| TEXAS INSTRUMENTS INCORPORATED
| Standard Linear and Logic Group
| IBIS Model of SN74ACT244
| OCTAL BUFFERS/DRIVERS WITH 3-STATE OUTPUTS
| This file contains package information for the following:
|  SSOP 20-pin (DB) package as [Component] ACT244A_DB
|  SOIC 20-pin (DW) package as [Component] ACT244A_DW
|  PDIP 20-pin (N) package as [Component] ACT244A_N
|  SOP 20-pin (NS) package as [Component] ACT244A_NS
|  TSSOP 20-pin (PW) package as [Component] ACT244A_PW
| This device can be powered at the following Vccs:
|  5 volt Vcc
| This file provides unique models under the [Model Selector] for each Vcc.
| For operation at a specific Vcc, select the appropriate model after each
| [Model Selector] keyword.
[IBIS Ver]   3.2
[Comment char]  |_char
[File Name]   sn74act244.ibs
[File Rev]   1.2 | a_die
[Date]   September 02, 2003
[Source]   Data created from TI-SPICE simulations at TI-SLL.
[Notes]   The following is an IBIS list for the ACT244A.
   Please contact sllibis@ti.com with questions and
   comments concerning SLL IBIS models.
   This IBIS model is created from a BA (back annotated netlist)
[Disclaimer] Property of Texas Instruments Incorporated.  Unauthorized
   reproduction and/or distribution is strictly prohibited.
   This product is protected under copyright law.
   Created  2003, (C) Copyright  2003, Texas Instruments
   Incorporated, All Rights Reserved
   UNLESS THERE IS A SIGNED, WRITTEN AGREEMENT TO THE
   CONTRARY, TEXAS INSTRUMENTS (TI) IS PROVIDING THE IBIS
   MODELS  AND WITHOUT ANY WARRANTY, EXPRESSED OR
   IMPLIED.  TI assumes no liability for:
   1) the accuracy of the IBIS models provided to your
   company;
   2) the proper functioning of these IBIS Models in your
   design or for any resulting applications; or
   3) infringement of patents, copyrights or intellectual
   property rights resulting from your use of these IBIS
   models.
   TI provides IBIS Models as a service to our customers.
   You and your company shall not distribute, sell or give
   these models to anyone else without prior written
   permission from TI.
   TI reserves the right to make changes to our products or
   to discontinue any semiconductor product or service
   without notice, and advises our customers to obtain the
   latest version of relevant information to verify, before
   placing orders, that the information being relied on is
   current.
   Please be aware that your receipt and use of the IBIS
   information provided shall serve as acceptance of these
   terms and conditions.  If you do not accept these terms,
   you should return or destroy the IBIS models and any
   other accompanying information immediately.
| Component ACT244A_DB 20-pin SSOP
[Component]   ACT244A_DB
[Manufacturer]   Texas Instruments, Inc.
[Package]
|   typ   min   max
R_pkg   4.000e-02   3.500e-02   5.100e-02
L_pkg   3.495e-09   3.035e-09   4.314e-09
C_pkg   4.200e-13   3.460e-13   5.020e-13
[Pin]   signal_name   model_name   R_pin   L_pin   C_pin
1   1NOE   ACT244_NOE   4.900e-02   4.310e-09   5.020e-13
2   1A1   ACT244_IN   4.800e-02   3.903e-09   4.870e-13
3   2Y4   ACT244_OUT   3.500e-02   3.189e-09   3.960e-13
4   1A2   ACT244_IN   3.500e-02   3.036e-09   3.470e-13
5   2Y3   ACT244_OUT   3.500e-02   3.035e-09   3.670e-13
6   1A3   ACT244_IN   3.500e-02   3.035e-09   3.670e-13
7   2Y2   ACT244_OUT   3.500e-02   3.036e-09   3.470e-13
8   1A4   ACT244_IN   3.500e-02   3.189e-09   3.970e-13
9   2Y1   ACT244_OUT   4.700e-02   3.899e-09   4.880e-13
10   GND   GND   5.100e-02   4.314e-09   5.000e-13
11   2A1   ACT244_IN   5.100e-02   4.314e-09   5.000e-13
12   1Y4   ACT244_OUT   4.700e-02   3.899e-09   4.880e-13
13   2A2   ACT244_IN   3.500e-02   3.189e-09   3.970e-13
14   1Y3   ACT244_OUT   3.500e-02   3.036e-09   3.460e-13
15   2A3   ACT244_IN   3.500e-02   3.035e-09   3.670e-13
16   1Y2   ACT244_OUT   3.500e-02   3.035e-09   3.670e-13
17   2A4   ACT244_IN   3.500e-02   3.036e-09   3.460e-13
18   1Y1   ACT244_OUT   3.500e-02   3.189e-09   3.970e-13
19   2NOE   ACT244_NOE   4.700e-02   3.899e-09   4.880e-13
20   VCC   POWER   5.100e-02   4.314e-09   5.020e-13
| Component ACT244A_DW 20-pin SOIC
[Component]   ACT244A_DW
[Manufacturer]   Texas Instruments, Inc.
[Package]
|   typ   min   max
R_pkg   3.800e-02   3.300e-02   4.500e-02
L_pkg   5.012e-09   4.110e-09   6.349e-09
C_pkg   7.170e-13   5.300e-13   8.680e-13
[Pin]   signal_name   model_name   R_pin   L_pin   C_pin
1   1NOE   ACT244_NOE   4.200e-02   6.336e-09   8.650e-13
2   1A1   ACT244_IN   4.300e-02   5.542e-09   8.670e-13
3   2Y4   ACT244_OUT   3.400e-02   4.714e-09   7.320e-13
4   1A2   ACT244_IN   3.400e-02   4.377e-09   5.910e-13
5   2Y3   ACT244_OUT   3.600e-02   4.130e-09   5.330e-13
6   1A3   ACT244_IN   3.500e-02   4.111e-09   5.300e-13
7   2Y2   ACT244_OUT   3.400e-02   4.284e-09   5.830e-13
8   1A4   ACT244_IN   3.400e-02   4.634e-09   7.260e-13
9   2Y1   ACT244_OUT   4.000e-02   5.518e-09   8.650e-13
10   GND   GND   4.300e-02   6.349e-09   8.660e-13
11   2A1   ACT244_IN   4.100e-02   6.281e-09   8.610e-13
12   1Y4   ACT244_OUT   4.500e-02   5.561e-09   8.680e-13
13   2A2   ACT244_IN   3.300e-02   4.778e-09   7.420e-13
14   1Y3   ACT244_OUT   3.500e-02   4.414e-09   5.960e-13
15   2A3   ACT244_IN   3.500e-02   4.110e-09   5.330e-13
16   1Y2   ACT244_OUT   3.600e-02   4.130e-09   5.330e-13
17   2A4   ACT244_IN   3.400e-02   4.377e-09   5.910e-13
18   1Y1   ACT244_OUT   3.400e-02   4.714e-09   7.310e-13
19   2NOE   ACT244_NOE   4.300e-02   5.569e-09   8.680e-13
20   VCC   POWER   4.200e-02   6.308e-09   8.640e-13
| Component ACT244A_N 20-pin PDIP
[Component]   ACT244A_N
[Manufacturer]   Texas Instruments, Inc.
[Package]
|   typ   min   max
R_pkg   4.300e-02   3.800e-02   5.000e-02
L_pkg   7.384e-09   4.680e-09   1.032e-08
C_pkg   5.100e-13   2.310e-13   8.210e-13
[Pin]   signal_name   model_name   R_pin   L_pin   C_pin
1   1NOE   ACT244_NOE   4.200e-02   9.427e-09   8.100e-13
2   1A1   ACT244_IN   4.600e-02   8.544e-09   4.560e-13
3   2Y4   ACT244_OUT   4.800e-02   7.163e-09   4.350e-13
4   1A2   ACT244_IN   4.000e-02   4.825e-09   2.610e-13
5   2Y3   ACT244_OUT   4.000e-02   5.284e-09   6.480e-13
6   1A3   ACT244_IN   4.000e-02   4.686e-09   2.320e-13
7   2Y2   ACT244_OUT   4.000e-02   6.359e-09   4.890e-13
8   1A4   ACT244_IN   3.800e-02   7.982e-09   4.750e-13
9   2Y1   ACT244_OUT   4.300e-02   9.403e-09   4.750e-13
10   GND   GND   5.000e-02   1.032e-08   8.050e-13
11   2A1   ACT244_IN   5.000e-02   1.028e-08   8.100e-13
12   1Y4   ACT244_OUT   4.300e-02   9.383e-09   4.770e-13
13   2A2   ACT244_IN   3.800e-02   7.978e-09   4.760e-13
14   1Y3   ACT244_OUT   4.000e-02   6.302e-09   4.920e-13
15   2A3   ACT244_IN   4.000e-02   4.680e-09   2.310e-13
16   1Y2   ACT244_OUT   4.000e-02   5.284e-09   6.480e-13
17   2A4   ACT244_IN   4.000e-02   4.822e-09   2.610e-13
18   1Y1   ACT244_OUT   4.700e-02   7.118e-09   4.390e-13
19   2NOE   ACT244_NOE   4.600e-02   8.492e-09   4.610e-13
20   VCC   POWER   4.300e-02   9.348e-09   8.210e-13
| Component ACT244A_NS 20-pin SOP
[Component]   ACT244A_NS
[Manufacturer]   Texas Instruments, Inc.
[Package]
|   typ   min   max
R_pkg   4.400e-02   2.900e-02   5.800e-02
L_pkg   3.666e-09   2.317e-09   5.115e-09
C_pkg   5.480e-13   3.160e-13   7.250e-13
[Pin]   signal_name   model_name   R_pin   L_pin   C_pin
1   1NOE   ACT244_NOE   5.800e-02   5.115e-09   7.250e-13
2   1A1   ACT244_IN   5.300e-02   4.591e-09   7.240e-13
3   2Y4   ACT244_OUT   4.900e-02   3.754e-09   5.720e-13
4   1A2   ACT244_IN   2.900e-02   2.549e-09   3.880e-13
5   2Y3   ACT244_OUT   3.100e-02   2.317e-09   3.160e-13
6   1A3   ACT244_IN   3.100e-02   2.317e-09   3.160e-13
7   2Y2   ACT244_OUT   2.900e-02   2.556e-09   3.990e-13
8   1A4   ACT244_IN   4.900e-02   3.754e-09   5.790e-13
9   2Y1   ACT244_OUT   5.300e-02   4.591e-09   7.240e-13
10   GND   GND   5.800e-02   5.115e-09   7.250e-13
11   2A1   ACT244_IN   5.800e-02   5.115e-09   7.250e-13
12   1Y4   ACT244_OUT   5.300e-02   4.591e-09   7.240e-13
13   2A2   ACT244_IN   4.900e-02   3.754e-09   5.790e-13
14   1Y3   ACT244_OUT   2.900e-02   2.557e-09   3.990e-13
15   2A3   ACT244_IN   3.100e-02   2.317e-09   3.160e-13
16   1Y2   ACT244_OUT   3.100e-02   2.317e-09   3.160e-13
17   2A4   ACT244_IN   2.900e-02   2.557e-09   3.990e-13
18   1Y1   ACT244_OUT   4.900e-02   3.754e-09   5.790e-13
19   2NOE   ACT244_NOE   5.300e-02   4.591e-09   7.240e-13
20   VCC   POWER   5.800e-02   5.115e-09   7.250e-13
| Component ACT244A_PW 20-pin TSSOP
[Component]   ACT244A_PW
[Manufacturer]   Texas Instruments, Inc.
[Package]
|   typ   min   max
R_pkg   5.000e-02   4.200e-02   6.000e-02
L_pkg   2.802e-09   2.248e-09   3.553e-09
C_pkg   3.170e-13   2.020e-13   4.430e-13
[Pin]   signal_name   model_name   R_pin   L_pin   C_pin
1   1NOE   ACT244_NOE   5.500e-02   3.461e-09   4.400e-13
2   1A1   ACT244_IN   5.500e-02   3.150e-09   4.010e-13
3   2Y4   ACT244_OUT   4.200e-02   2.619e-09   3.020e-13
4   1A2   ACT244_IN   4.500e-02   2.273e-09   2.020e-13
5   2Y3   ACT244_OUT   4.500e-02   2.248e-09   2.240e-13
6   1A3   ACT244_IN   4.500e-02   2.273e-09   2.260e-13
7   2Y2   ACT244_OUT   4.400e-02   2.323e-09   2.050e-13
8   1A4   ACT244_IN   4.600e-02   2.704e-09   3.070e-13
9   2Y1   ACT244_OUT   6.000e-02   3.265e-09   4.110e-13
10   GND   GND   5.700e-02   3.506e-09   4.360e-13
11   2A1   ACT244_IN   5.800e-02   3.553e-09   4.370e-13
12   1Y4   ACT244_OUT   5.800e-02   3.193e-09   4.050e-13
13   2A2   ACT244_IN   4.200e-02   2.704e-09   3.110e-13
14   1Y3   ACT244_OUT   4.600e-02   2.392e-09   2.100e-13
15   2A3   ACT244_IN   4.700e-02   2.334e-09   2.290e-13
16   1Y2   ACT244_OUT   4.700e-02   2.300e-09   2.270e-13
17   2A4   ACT244_IN   4.700e-02   2.349e-09   2.070e-13
18   1Y1   ACT244_OUT   4.500e-02   2.677e-09   3.060e-13
19   2NOE   ACT244_NOE   6.000e-02   3.235e-09   4.060e-13
20   VCC   POWER   5.600e-02   3.487e-09   4.430e-13
| Models and submodels in the file (3): ACT244_IN (Input), ACT244_NOE (Input), ACT244_OUT (3-state)
